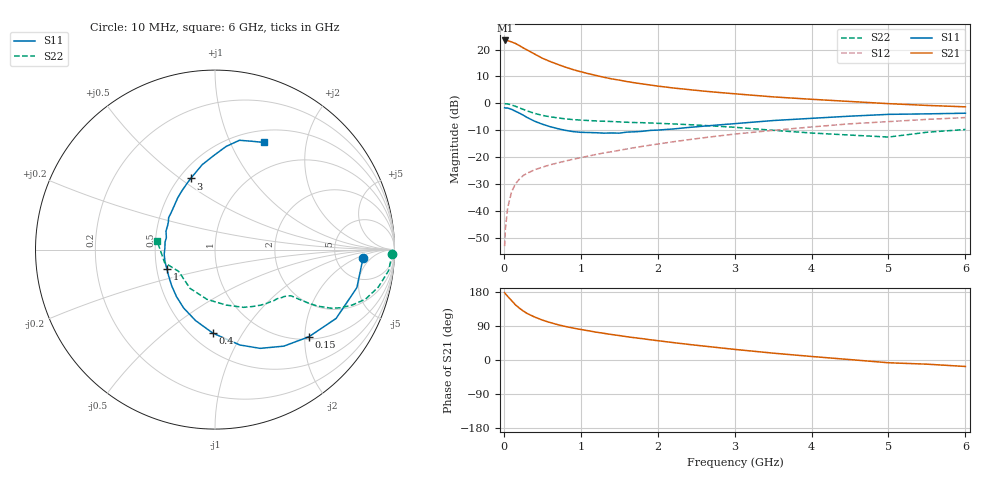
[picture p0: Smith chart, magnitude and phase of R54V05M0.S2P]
! SIEMENS Small Signal Semiconductors
! BFR183
! Si NPN RF Bipolar Junction Transistor in SOT23
! VCE = 4 V  IC = 5 mA
! Common Emitter S-Parameters:  May  1996
# GHz  S  MA  R  50
!  f  S11  S21  S12  S22
! GHz  MAG  ANG  MAG  ANG  MAG  ANG  MAG  ANG
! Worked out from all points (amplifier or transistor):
!   36 points, 10 MHz to 6 GHz, reference 50 ohm
!   highest |S21| = 23.4 dB at 20 MHz (marker M1)
!   |S21| within 3 dB of that: start of sweep to 267.3 MHz
!   unconditionally stable (mu >= 1): 1.038 GHz to 2.629 GHz
!   at 250 MHz: K = 0.41, MSG = 23.8 dB, |S12| = -26.9 dB
!   at 1.4 GHz: K = 1.06, MAG = 12.1 dB, |S12| = -18.0 dB
!   at 6 GHz: K = 0.88, MSG = 2.0 dB, |S12| = -5.3 dB
!   lowest NFmin = 1.15 dB at 450 MHz
!   S11 on the Smith chart (normalised r, x): 10 MHz: 10, -3; 150 MHz: 1.06, -2.10; 400 MHz: 0.63, -0.75; 1 GHz: 0.57, -0.14; 3 GHz: 0.57, +0.55; 6 GHz: 0.64, +1.34
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0.01  0.8278 -3.1  14.66 177.7  0.0022 90.1  0.9891 -1.3
0.02  0.8211 -6.1  14.81 174.9  0.0046 84.5  0.9828 -2.7
0.05  0.8184 -15.0  14.73 167.9  0.0114 83.4  0.975 -6.8
0.1  0.7762 -29.6  13.89 156.9  0.0225 75.1  0.934 -12.9
0.15  0.7137 -42.9  13.05 145.7  0.0316 69.3  0.8832 -18.2
0.2  0.6607 -54.5  11.92 137.3  0.0387 64.7  0.826 -21.9
0.25  0.6052 -65.4  10.81 129.7  0.0452 61.8  0.7749 -24.7
0.3  0.5492 -75.4  9.9 123.1  0.0498 59.8  0.7276 -26.7
0.4  0.4654 -91.5  8.274 113.4  0.0581 56.4  0.651 -28.9
0.5  0.4097 -105.4  6.926 105.4  0.0649 55.6  0.5977 -29.8
0.6  0.3691 -118.3  6.026 99.0  0.0717 55.4  0.5636 -30.3
0.7  0.3386 -129.3  5.316 93.3  0.078 56.0  0.5365 -30.7
0.8  0.3149 -139.9  4.718 88.5  0.0844 56.2  0.5149 -31.0
1  0.2893 -157.6  3.875 80.6  0.0974 57.6  0.4884 -31.8
1.1  0.2868 -166.8  3.565 77.1  0.1046 58.0  0.4792 -32.8
1.6  0.2919 159.3  2.546 61.4  0.1417 58.9  0.4451 -37.6
2.2  0.3335 132.9  1.935 46.0  0.1928 57.2  0.4143 -46.5
3  0.4191 108.8  1.508 28.0  0.268 51.1  0.3589 -63.7
3.5  0.4789 98.5  1.32 18.1  0.3147 45.7  0.3151 -78.7
4.5  0.5777 83.9  1.084 1.1  0.4164 34.1  0.257 -122.8
5.5  0.6377 71.2  0.916 -11.0  0.5033 21.5  0.2899 -165.4
6  0.6556 65.6  0.862 -17.1  0.544 13.4  0.3266 171.3
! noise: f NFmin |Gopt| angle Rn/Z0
0.45  1.15  0.25  40  0.26
0.9  1.2  0.25  93  0.22
1.8  1.95  0.32  170  0.13
